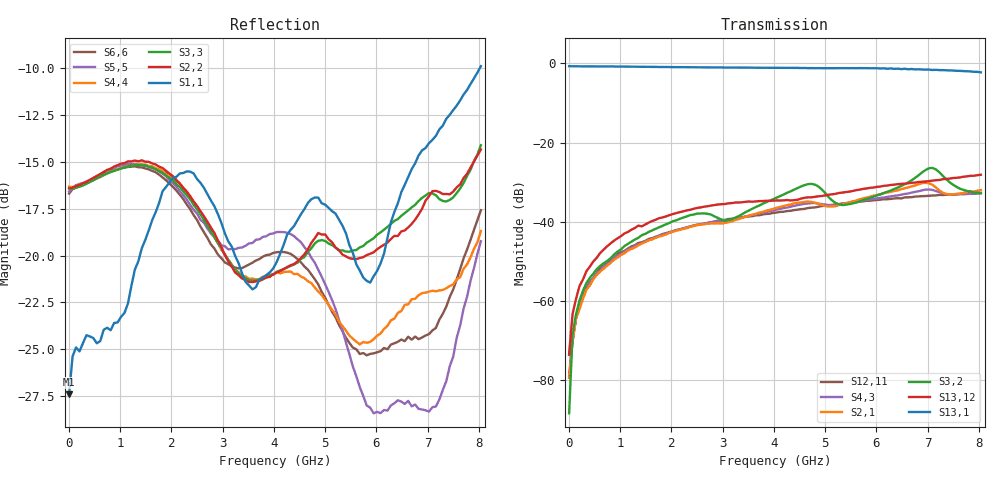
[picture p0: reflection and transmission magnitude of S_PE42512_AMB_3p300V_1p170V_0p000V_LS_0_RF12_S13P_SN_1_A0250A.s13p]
! Device ID: PE42512
! File Path: z:\PE42512\TE_GND_Post_Char_S-Param\All Parts\AMB\3p300\LS_0_RF12\PE42512_AMB_3p300V_1p170V_0p000V_LS_0_RF12_S13P_SN_1_A0250A.s13p
! Serial: 1
! Lot: A0250A
! Temp: AMB
! VDD: 3.300
! VSS: 0.000
! Control_Hi: 1.170
! Control_Lo: 0.000
! Logic State: LS_0_RF12
! Port 1:
! Port 2:
! Port 3:
! Port 4:
! Port 5:
! Port 6:
! Port 7:
! Port 8:
! Port 9:
! Port 10:
! Port 11:
! Port 12:
! Port 13:
! ThroughPath:1-13
! IDD: 0.0001077521
! ISS/IDD2: 4.29e-008
! IDMM3/IDD3: -2.078e-007
! Comment:
#  Hz  S  RI  R  50
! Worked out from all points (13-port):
!   120 points, 10 MHz to 8.037 GHz, reference 50 ohm
!   strongest paths, dB at 10 MHz, 2.034 GHz, 4.057 GHz, 6.08 GHz, 8.037 GHz:
!     S13,1: -0.7, -0.9, -1.1, -1.3, -2.2
!     S13,12: -73.3, -38.0, -34.6, -31.1, -28.1
!     S3,2: -88.4, -39.9, -33.9, -33.0, -32.7
!     S2,1: -79.4, -42.5, -36.5, -33.1, -32.0
!     S4,3: -78.9, -42.4, -36.9, -34.0, -32.8
!     S12,11: -73.6, -42.4, -37.7, -34.4, -32.7
!   lowest |S11| = -27.4 dB at 10 MHz (marker M1), VSWR 1.09, Z = 53 - j3.25 ohm
!   |S11| at or under -10 dB: start of sweep to 8.022 GHz
